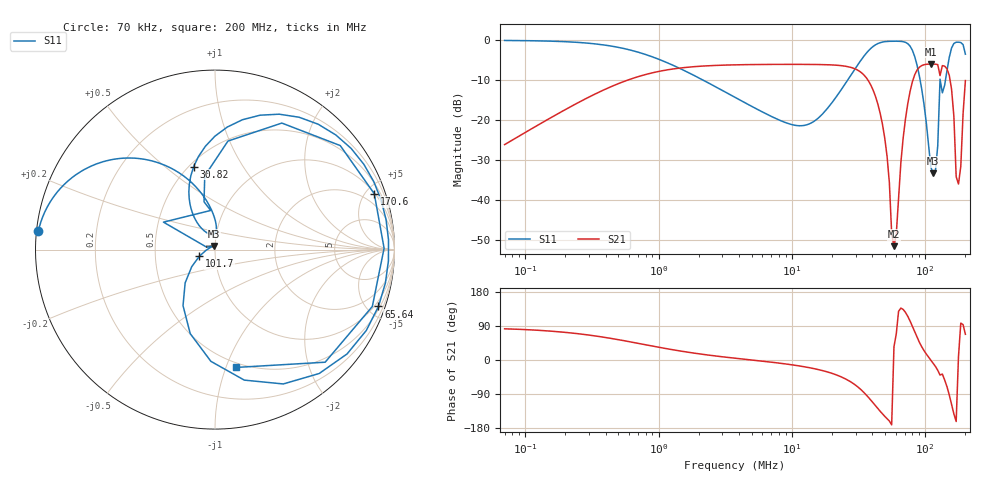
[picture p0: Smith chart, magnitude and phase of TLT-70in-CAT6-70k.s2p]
! ListType=Log
!!70in CAT-6 TP ID=1in 20T 1:4 TLT
# MHZ S RI R 50
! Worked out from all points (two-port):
!   201 points, 70 kHz to 200 MHz, reference 50 ohm
!   highest |S21| = -5.98 dB at 110.1 MHz (marker M1); lowest = -51.5 dB at 58.26 MHz (marker M2)
!   |S21| within 3 dB of the highest: 727.6 kHz to 35.24 MHz (34.51 MHz wide, 192 % of centre); 82.76 MHz to 151.7 MHz (68.94 MHz wide, 58.8 % of centre)
!   lowest |S11| = -33.2 dB at 114.6 MHz (marker M3), VSWR 1.04, Z = 49.2 + j2.01 ohm
!   |S11| at or under -10 dB: 2.158 MHz to 26.17 MHz (24.02 MHz wide, 170 % of centre); 91.52 MHz to 129 MHz (37.51 MHz wide, 34 % of centre); 129.5 MHz to 141.8 MHz (12.3 MHz wide, 9.07 % of centre)
!   S12 and S22 are empty: the file has one direction only
!   S11 on the Smith chart (normalised r, x): 70 kHz: 0.01, +0.05; 30.82 MHz: 0.53, +0.63; 65.64 MHz: 0.65, -5.85; 101.7 MHz: 0.84, -0.06; 170.6 MHz: 1.06, +5.69; 200 MHz: 0.46, -1.09
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0.07  -0.9843 0.1016  0.00664 0.0491  0 0  0 0
0.2707737  -0.8612 0.3411  0.0672 0.1647  0 0  0 0
1.00655  -0.3126 0.4826  0.339 0.2247  0 0  0 0
3.741657  -0.00802 0.1926  0.4893 0.0403  0 0  0 0
14.47346  -0.0356 0.0887  0.459 -0.1889  0 0  0 0
30.82379  -0.1186 0.463  0.1483 -0.3986  0 0  0 0
44.09638  0.5747 0.6987  -0.0979 -0.1252  0 0  0 0
53.80235  0.9259 0.2751  -0.0157 -0.00541  0 0  0 0
58.25867  0.9667 0.0546  0.00219 0.00153  0 0  0 0
65.64468  0.9107 -0.3169  -0.0217 0.0203  0 0  0 0
80.0936  0.1633 -0.7272  0.0069 0.302  0 0  0 0
101.6894  -0.0872 -0.0371  0.479 0.1379  0 0  0 0
110.1121  -0.0218 0.0139  0.5026 -0.00395  0 0  0 0
114.5816  -0.00757 0.0204  0.4969 -0.0739  0 0  0 0
124.0721  -0.0461 0.0133  0.4396 -0.2251  0 0  0 0
129.1082  -0.2871 0.1529  0.2771 -0.2308  0 0  0 0
134.3487  -0.0241 0.2181  0.3824 -0.2899  0 0  0 0
151.3814  0.0722 0.6047  -0.0134 -0.3632  0 0  0 0
163.9199  0.6977 0.5796  -0.0886 -0.0687  0 0  0 0
170.5734  0.8875 0.3111  -0.0188 -0.00598  0 0  0 0
184.7016  0.8766 -0.3168  -0.00339 0.0263  0 0  0 0
200  0.1191 -0.6564  0.1178 0.2891  0 0  0 0
